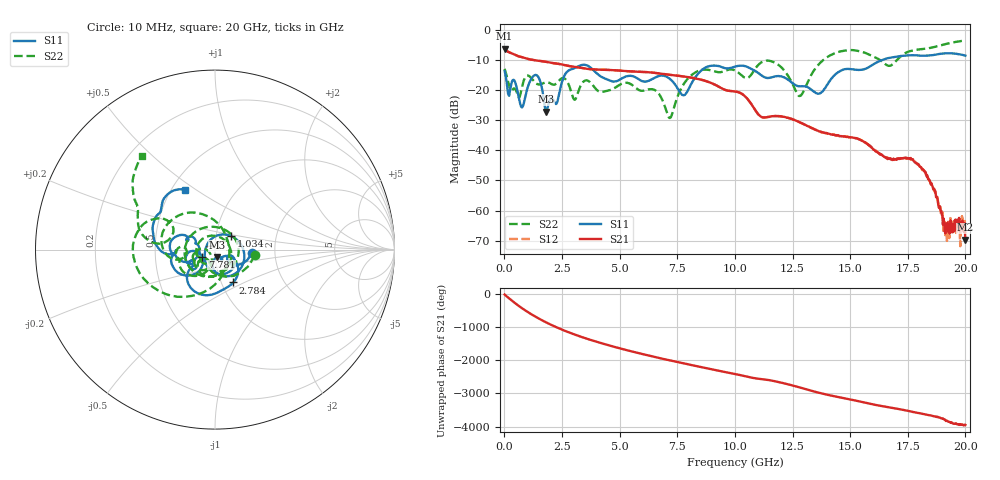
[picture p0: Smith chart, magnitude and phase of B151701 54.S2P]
!  2-Port S-parameters saved by WinCal
! VAR MeasName=S-Parameters (CALIBRATED_DATA) read from VNA (N5244A)
! VAR MeasDate=2015-12-24 19:16:15
! VAR NAME=B151701 54
! VAR FILENAME=B151701 54.S2P
! VAR DATE=2015-12-24 19:16:15
! VAR PHYS_PORTS=1,3
# Hz S DB R 50
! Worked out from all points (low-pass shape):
!   801 points, 10 MHz to 20 GHz, reference 50 ohm
!   highest |S21| = -6.27 dB at 10 MHz (marker M1); lowest = -69.7 dB at 20 GHz (marker M2)
!   |S21| within 3 dB of the highest: start of sweep to 828.8 MHz
!   lowest |S11| = -27.2 dB at 1.809 GHz (marker M3), VSWR 1.09, Z = 50.9 - j4.34 ohm
!   |S11| at or under -10 dB: start of sweep to 16.41 GHz
!   |S22| runs from -29.3 to -3.6 dB; largest |S21 - S12| = 0.0016
!   S11 on the Smith chart (normalised r, x): 10 MHz: 1.51, -0.07; 1.034 GHz: 1.18, +0.18; 2.784 GHz: 1.14, -0.44; 7.781 GHz: 0.86, -0.07; 20 GHz: 0.59, +0.45
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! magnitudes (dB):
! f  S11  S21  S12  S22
! 10 MHz  -13.8  -6.3  -6.2  -13.0
! 759.6 MHz  -25.8  -9.1  -9.1  -19.1
! 1.034 GHz  -18.6  -9.7  -9.7  -15.3
! 1.434 GHz  -15.3  -10.2  -10.2  -18.1
! 1.809 GHz  -27.2  -10.7  -10.7  -17.5
! 2.784 GHz  -13.6  -12.0  -12.0  -18.1
! 3.058 GHz  -12.7  -12.3  -12.3  -23.2
! 3.358 GHz  -11.7  -12.7  -12.7  -17.9
! 6.682 GHz  -15.4  -14.5  -14.5  -21.1
! 7.181 GHz  -16.4  -15.0  -15.0  -29.3
! 7.781 GHz  -21.8  -15.5  -15.6  -18.0
! 8.706 GHz  -12.6  -17.0  -16.9  -13.2
! 10.01 GHz  -12.3  -20.5  -20.5  -13.5
! 11.63 GHz  -15.7  -28.7  -28.7  -10.6
! 12.8 GHz  -18.8  -30.6  -30.7  -22.0
! 13.35 GHz  -20.1  -32.7  -32.7  -14.4
! 14.88 GHz  -13.0  -35.5  -35.6  -6.8
! 16.68 GHz  -9.4  -42.7  -42.9  -12.0
! 17.98 GHz  -8.6  -44.7  -45.0  -6.5
! 18.7 GHz  -8.3  -53.6  -54.3  -5.7
! 19.13 GHz  -7.9  -67.6  -65.4  -4.8
! 20 GHz  -8.6  -69.7  -67.5  -3.6
